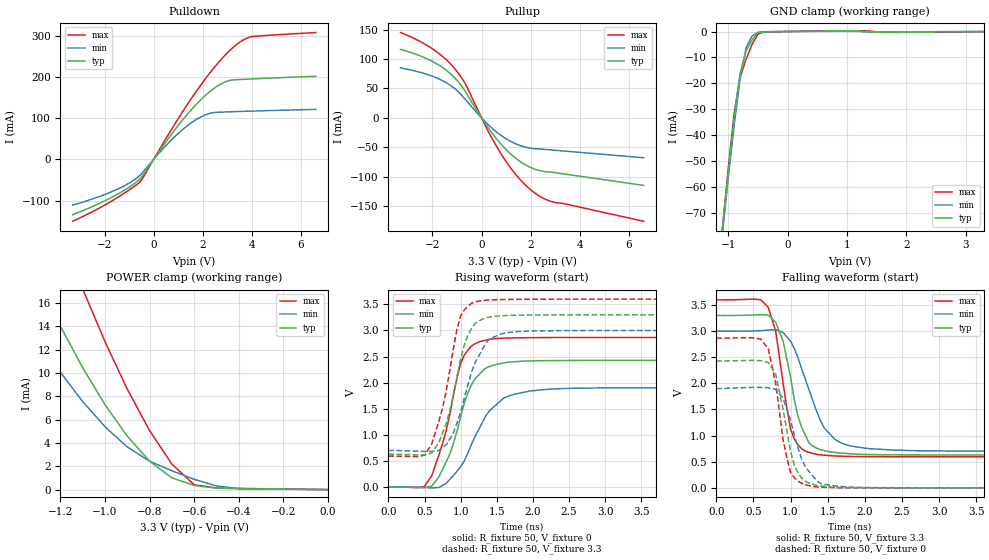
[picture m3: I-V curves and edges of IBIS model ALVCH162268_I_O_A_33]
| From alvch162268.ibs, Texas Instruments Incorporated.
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|************* ALVCH162268 OUTPUT (3.3 V) MODEL**************
[Model]   ALVCH162268_I_O_A_33
Model_type  I/O
Polarity   Non-Inverting
Enable   Active-Low
Vinl = 0.8V
Vinh = 2.0V
Vmeas = 1.5V
Cref = 50pF
Rref = 500
Vref = 0
| variable   typ   min   max
C_comp   8.15pF   NA   NA
[Temperature Range]   50   100   0
[Voltage range]   3.3   3   3.6
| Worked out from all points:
|   slope of the pulldown table from 0 to 0.495 V, typ, clamps not added: 11.7 ohm
|   slope of the pullup table from 0 to 0.495 V, typ, clamps not added: 16.7 ohm
|   GND clamp passes 1 mA (typ) near -0.52 V on its own axis
|   POWER clamp passes 1 mA (typ) near -0.70 V on its own axis
|   rising waveform, R_fixture 50, V_fixture 0: 20-80 % time 344ps typ, 453ps min, 297ps max; typ from 0 V to 2.43 V
|   falling waveform, R_fixture 50, V_fixture 3.3: 20-80 % time 243ps typ, 361ps min, 192ps max; typ from 3.3 V to 0.629 V
|   rising waveform, R_fixture 50, V_fixture 3.3: 20-80 % time 278ps typ, 331ps min, 262ps max; typ from 0.629 V to 3.3 V
|   falling waveform, R_fixture 50, V_fixture 0: 20-80 % time 206ps typ, 264ps min, 195ps max; typ from 2.43 V to 0 V
|Process range|   weak   strong
[Pullup]
|   50C:3.3V:   100C:3V:weak   0C:3.6V:strong
|   Voltage   I(typ)   I(min)   I(max)
-3.3V     116.5mA    84.95mA    145.1mA
-2V       95.96mA    70.81mA    117.4mA
-1.5V     82.97mA    61.22mA    101.3mA
-1.1V     68.45mA    50.02mA    84.05mA
-600mV    40.58mA    28.42mA    53.02mA
200mV     -12.69mA   -8.672mA   -17mA
700mV     -40.26mA   -26.91mA   -54.82mA
1.4V      -68.97mA   -44.29mA   -96.68mA
2.1V      -86.16mA   -52.15mA   -125.6mA
2.5V      -90.83mA   -53.35mA   -136.4mA
2.9V      -92.65mA   -54.76mA   -142.9mA
6.6V      -114.8mA   -67.85mA   -175.9mA
[Pulldown]
|   50C:3.3V:   100C:3V:weak   0C:3.6V:strong
|   Voltage   I(typ)   I(min)   I(max)
-3.3V     -134.3mA   -111.2mA   -150.4mA
-1.5V     -85.64mA   -73.09mA   -93.67mA
-900mV    -63.57mA   -54.24mA   -70.08mA
-500mV    -43.85mA   -35.33mA   -50.71mA
700mV     58.96mA    45.81mA    70.18mA
1.7V      131.3mA    95.43mA    162mA
2.2V      160.2mA    110mA      203mA
2.6V      178.2mA    114.4mA    232.6mA
3V        190mA      115.3mA    258.6mA
3.4V      193.6mA    116.1mA    279.9mA
4V        195.3mA    117.2mA    298.2mA
6.6V      201.7mA    121.4mA    307.9mA
[GND Clamp]
|   50C:3.3V:   100C:3V:weak   0C:3.6V:strong
|   Voltage   I(typ)   I(min)   I(max)
-3.3V     -639mA     -614.4mA   -663.6mA
-1.1V     -77.02mA   -78.47mA   -76.68mA
-1V       -54.25mA   -56.74mA   -52.94mA
-900mV    -33.14mA   -36.27mA   -31.65mA
-800mV    -16.15mA   -18.34mA   -17.68mA
-700mV    -7.612mA   -6.307mA   -10.76mA
-600mV    -3.323mA   -1.797mA   -5.038mA
-500mV    -470.1uA   -328.9uA   -1.041mA
-400mV    -109.7uA   -99.57uA   -141.7uA
700mV     155.2uA    101.7uA    211.8uA
1.6V      -218.7uA   -130.5uA   -322.9uA
3.3V      159.2pA    44.74uA    -73.47uA
[POWER Clamp]
|   50C:3.3V:   100C:3V:weak   0C:3.6V:strong
|   Voltage   I(typ)   I(min)   I(max)
-3.3V     130.3mA    99.71mA    165.8mA
-1.5V     26.54mA    19.28mA    38.52mA
-1.4V     22.09mA    15.96mA    32.77mA
-1.3V     17.9mA     12.87mA    27.28mA
-1.2V     14mA       10.05mA    22.07mA
-1.1V     10.44mA    7.537mA    17.18mA
-900mV    4.574mA    3.653mA    8.601mA
-800mV    2.435mA    2.435mA    5.059mA
-700mV    1.009mA    1.617mA    2.181mA
-600mV    360.1uA    881.6uA    415.4uA
-400mV    82.07uA    82.05uA    103.7uA
0V        154.3pA    691.3pA    84.99pA
[ramp]
| variable   typ   min   max
dV/dt_r   1.4628E+00/3.4670E-10  1.1492E+00/4.5671E-10  1.7244E+00/2.9843E-10
dV/dt_f   1.6116E+00/2.4356E-10  1.3968E+00/3.6198E-10  1.8100E+00/1.8919E-10
[Rising Waveform]
R_fixture = 50
V_fixture = 0
V_fixture_min = 0
V_fixture_max = 0
C_fixture = 0
L_fixture = 0
|   50C:3.3V:   100C:3V:weak   0C:3.6V:strong
|   Time   V(typ)   V(min)   V(max)
0s        0V         0V         0V
500ps     -10.41mV   -6.146mV   15.13mV
600ps     20.37mV    -12.47mV   219.3mV
750ps     343.5mV    35.49mV    837.2mV
1ns       1.352V     391.5mV    2.375V
1.15ns    1.961V     823.3mV    2.703V
1.4ns     2.311V     1.466V     2.833V
1.7ns     2.397V     1.762V     2.856V
2.45ns    2.425V     1.89V      2.865V
13.5ns    2.428V     1.903V     2.866V
[Falling Waveform]
R_fixture = 50
V_fixture = 3.3
V_fixture_min = 3
V_fixture_max = 3.6
C_fixture = 0
L_fixture = 0
|   50C:3.3V:   100C:3V:weak   0C:3.6V:strong
|   Time   V(typ)   V(min)   V(max)
0s        3.3V       3V         3.6V
700ps     3.305V     3.02V      3.454V
800ps     3.168V     3.029V     2.995V
900ps     2.805V     2.971V     1.998V
1ns       2.114V     2.806V     1.121V
1.15ns    1.158V     2.277V     747mV
1.35ns    759.8mV    1.468V     641.2mV
1.65ns    669.4mV    882.5mV    607mV
2.4ns     632mV      721.9mV    595.6mV
13.5ns    629.3mV    701.1mV    595mV
[Rising Waveform]
R_fixture = 50
V_fixture = 3.3
V_fixture_min = 3
V_fixture_max = 3.6
C_fixture = 0
L_fixture = 0
|   50C:3.3V:   100C:3V:weak   0C:3.6V:strong
|   Time   V(typ)   V(min)   V(max)
0s        629.3mV    701.1mV    595mV
500ps     617mV      685.2mV    613.2mV
700ps     858mV      701mV      1.268V
850ps     1.468V     925.7mV    2.241V
1ns       2.458V     1.436V     3.275V
1.1ns     2.905V     1.959V     3.464V
1.25ns    3.181V     2.51V      3.561V
1.4ns     3.257V     2.839V     3.585V
1.95ns    3.295V     2.987V     3.597V
13.5ns    3.3V       3V         3.6V
[Falling Waveform]
R_fixture = 50
V_fixture = 0
V_fixture_min = 0
V_fixture_max = 0
C_fixture = 0
L_fixture = 0
|   50C:3.3V:   100C:3V:weak   0C:3.6V:strong
|   Time   V(typ)   V(min)   V(max)
0s        2.428V     1.903V     2.866V
600ps     2.434V     1.923V     2.848V
700ps     2.4V       1.916V     2.66V
800ps     2.177V     1.883V     2V
900ps     1.492V     1.713V     911.2mV
1ns       695.2mV    1.295V     292.3mV
1.15ns    185.5mV    548mV      86.44mV
1.3ns     68.78mV    224.6mV    25.74mV
2.1ns     1.711mV    4.034mV    883.6uV
13.5ns    204.9nV    -6.034uV   -171.4nV
